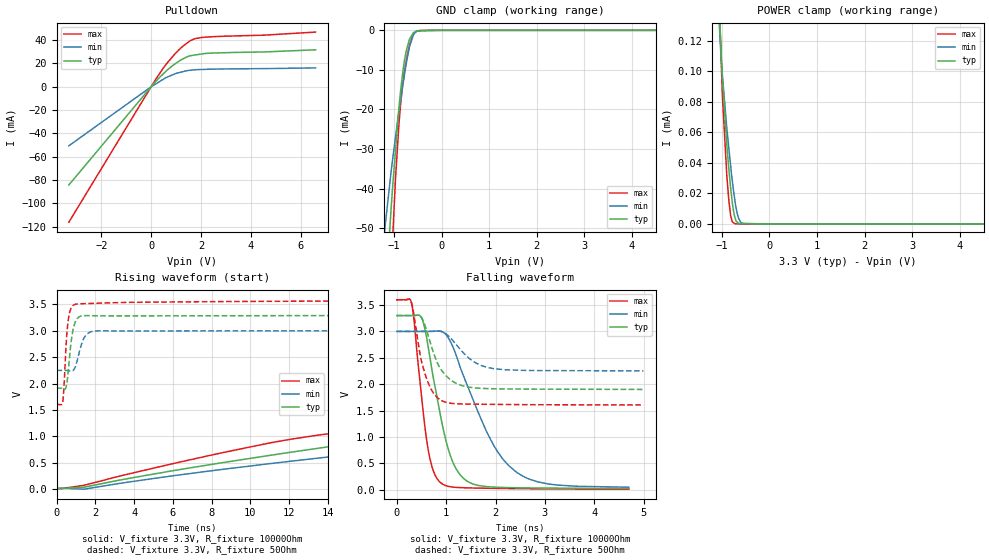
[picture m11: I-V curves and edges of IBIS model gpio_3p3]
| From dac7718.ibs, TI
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|   gpio_3p3 Model
[Model]   gpio_3p3
Model_type   I/O_open_drain
Polarity   Non-Inverting
Enable   Active-Low
Vinl = 0.6
Vinh = 2.3
Vmeas = 1.65
Vref = 3.3
Cref = 15pF
Rref = 10000
|   typ   min   max
|   (nom PVT)   (Fast PVT)   (slow PVT)
|C_comp from Frequency Method (F=50MHz)
|Average
|C_comp   3.710e-12   3.075e-12   4.212e-12
|OFF state: BUFFER IN HIGH IMPEDANCE
|C_comp   3.538e-12   2.912e-12   4.031e-12
|ON state : BUFFER OUTPUT TURNED LOW
C_comp   3.882e-12   3.237e-12   4.393e-12
|C_comp from LC Tank Method (L=1nH)
|Resonant Frequency(Hz)   3.01e9   3.17e9   2.88e9
|C_comp   2.799e-12   2.523e-12   3.057e-12
| Where nom  PVT is Nominal Process,  3.3V,  33C
|   Fast PVT is Strong Process,   3.6V,  -40C
|   Slow PVT is Weak Process,   3V,  113C
[Voltage Range]   3.3   3   3.6
[Temperature Range]   33   113   -40
[Pullup Reference]   3.3   3   3.6
[Pulldown Reference]   0   0   0
[Power Clamp Reference]   3.3   3   3.6
[GND Clamp Reference]   0   0   0
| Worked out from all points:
|   slope of the pulldown table from 0 to 0.495 V, typ, clamps not added: 44 ohm
|   GND clamp passes 1 mA (typ) near -0.61 V on its own axis
|   falling waveform, V_fixture 3.3V, R_fixture 10000Ohm: 20-80 % time 427ps typ, 851ps min, 259ps max; typ from 3.3 V to 0.025 V
|   rising waveform, V_fixture 3.3V, R_fixture 10000Ohm: 20-80 % time 145ns typ, 173ns min, 113ns max; typ from 0.013 V to 3.3 V
|   falling waveform, V_fixture 3.3V, R_fixture 50Ohm: 20-80 % time 374ps typ, 490ps min, 279ps max; typ from 3.3 V to 1.9 V
|   rising waveform, V_fixture 3.3V, R_fixture 50Ohm: 20-80 % time 260ps typ, 362ps min, 207ps max; typ from 1.91 V to 3.29 V
[Pulldown]
|   Voltage   I(typ)   I(min)   I(max)
-3.3V     -84.11mA   -50.56mA   -116mA
172.8mV   4.256mA    2.307mA    5.988mA
651.6mV   14.44mA    8.381mA    20.55mA
939.6mV   19.39mA    10.93mA    27.83mA
1.246V    23.59mA    12.82mA    34.29mA
1.573V    26.65mA    14.24mA    39.51mA
1.814V    27.44mA    14.64mA    41.5mA
2.012V    28.08mA    14.83mA    42.2mA
2.627V    29.05mA    15.19mA    43.08mA
4.5V      29.86mA    15.58mA    44.23mA
6.6V      31.7mA     16.21mA    46.9mA
[GND Clamp]
|   Voltage   I(typ)   I(min)   I(max)
-3.3V     -538.7mA   -365mA     -768.8mA
-1.188V   -68.37mA   -49.74mA   -97.51mA
-1.058V   -44.8mA    -35.49mA   -60.39mA
-1.026V   -39.32mA   -32.46mA   -52.23mA
-896.4mV  -19.67mA   -20.36mA   -23.81mA
-860.4mV  -15.3mA    -17.54mA   -18.7mA
-817.2mV  -10.85mA   -14.16mA   -13.74mA
-745.8mV  -5.372mA   -8.73mA    -7.971mA
-673.2mV  -2.23mA    -4.217mA   -3.715mA
-594mV    -629.8uA   -1.203mA   -1.026mA
-528mV    -157.1uA   -300.7uA   -246.8uA
6.6V      0A         0A         0A
[POWER Clamp]
|   Voltage   I(typ)   I(min)   I(max)
-3.3V     2.915mA    2.343mA    3.662mA
-1.069V   151.3uA    139.1uA    159.2uA
-1.023V   116.8uA    112.5uA    115.6uA
-990mV    96.18uA    97.69uA    84.41uA
-896.4mV  51.95uA    62.8uA     31.76uA
-853.2mV  35.78uA    49.58uA    15.18uA
-813.6mV  22.77uA    37.46uA    5.119uA
-778.8mV  13.28uA    27.7uA     1.37uA
-727.2mV  4.49uA     15.53uA    113.3nA
-648mV    306.3nA    3.616uA    0A
-567mV    237.2nA    417nA      0A
6.6V      0A         0A         0A
[Ramp]
R_load = 10000
|   typ   min   max
dV/dt_r   1.97221/1.45749e-07   1.78774/1.74761e-07   2.15396/1.12974e-07
dV/dt_f   1.97224/4.29349e-10   1.78827/8.66941e-10   2.15396/2.59254e-10
[Falling Waveform]
V_fixture = 3.3V
V_fixture_min = 3V
V_fixture_max = 3.6V
R_fixture = 10000Ohm
|   Time   V(typ)   V(min)   V(max)
0s        3.3V       3V         3.6V
300ps     3.3V       3V         3.533V
500ps     3.26V      3V         1.785V
620ps     2.8V       3V         852.8mV
880ps     1.431V     3.006V     141.1mV
1.1ns     609.2mV    2.783V     56.74mV
1.34ns    228.3mV    2.185V     39.92mV
1.96ns    52.07mV    848.8mV    28.17mV
2.42ns    39.6mV     337.9mV    22.84mV
4.7ns     25mV       48.97mV    12.67mV
[Rising Waveform]
V_fixture = 3.3V
V_fixture_min = 3V
V_fixture_max = 3.6V
R_fixture = 10000Ohm
|   Time   V(typ)   V(min)   V(max)
0s        12.93mV    19.54mV    10.06mV
12.12ns   701.5mV    531mV      948mV
22.04ns   1.146V     915.1mV    1.278V
34.06ns   1.372V     1.26V      1.498V
47.6ns    1.533V     1.449V     1.738V
121.4ns   2.32V      1.987V     2.874V
169ns     2.735V     2.289V     3.321V
224ns     3.056V     2.58V      3.503V
303ns     3.219V     2.837V     3.573V
581ns     3.296V     2.983V     3.6V
[Falling Waveform]
V_fixture = 3.3V
V_fixture_min = 3V
V_fixture_max = 3.6V
R_fixture = 50Ohm
|   Time   V(typ)   V(min)   V(max)
0s        3.3V       3V         3.6V
284ps     3.3V       3V         3.583V
484ps     3.286V     3V         2.506V
580ps     3.087V     3V         2.175V
742ps     2.6V       3.003V     1.835V
942ps     2.222V     2.985V     1.676V
1.188ns   2.024V     2.768V     1.631V
1.514ns   1.938V     2.456V     1.623V
1.94ns    1.915V     2.298V     1.619V
4.998ns   1.901V     2.253V     1.607V
[Rising Waveform]
V_fixture = 3.3V
V_fixture_min = 3V
V_fixture_max = 3.6V
R_fixture = 50Ohm
|   Time   V(typ)   V(min)   V(max)
0s        1.913V     2.249V     1.605V
320ps     1.91V      2.249V     1.655V
380ps     1.907V     2.249V     1.908V
490ps     1.933V     2.248V     2.702V
670ps     2.49V      2.241V     3.337V
820ps     2.954V     2.241V     3.466V
1.02ns    3.203V     2.373V     3.506V
1.41ns    3.286V     2.856V     3.513V
1.96ns    3.283V     2.995V     3.519V
30.39ns   3.294V     3V         3.586V
